| IBIS file stm32f373_378_383_lqfp100.ibs
[IBIS ver] 4.2
[File name] stm32f373_378_383_lqfp100.ibs
[File Rev] 1.0
[Date]  29-09-2025
[Source] Data Created at STMicroelectronics
[Notes]  File originated from ELDO simulations.
[Disclaimer]  This information is for modeling purpose only and is
   not guaranted. The information is subject to change without
   notice.
[Copyright] Copyright 2025 STMicroelectronics Inc.
|   Component stm32f373_378_383_lqfp100
[Component] stm32f373_378_383_lqfp100
[Manufacturer] STMicroelectronics
[Package]
| variable   typ   min   max
R_pkg  0  NA  NA
L_pkg  0  NA  NA
C_pkg  0  NA  NA
[Pin]   signal_name   model_name R_pin  L_pin C_pin
1 PE2 io8p_sudq_ft 0.132430474 7.03397E-09 1.35E-13
2 PE3 io8p_sudq_ft 0.133347678 6.76535E-09 1.95E-14
3 PE4 io8p_sudq_ft 0.12897311 6.4945E-09 1.04E-14
4 PE5 io8p_sudq_ft 0.125344562 6.20552E-09 5.24E-15
5 PE6 io8p_sudq_tc_v33 0.120515446 5.99116E-09 7.82E-15
6 VBAT POWER 0.12047071 5.94998E-09 6.53E-15
7 PC13 io8p_sudq_tc_v33 0.117880646 5.78336E-09 6.23E-15
8 PC14-OSC32_IN io8p_sudq_tc_v33 0.117278614 5.65387E-09 3.11E-15
9 PC15-OSC32_OUT io8p_sudq_tc_v33 0.11554812 5.54782E-09 1.39E-15
10 PF9 io8p_sudq_ft 0.114995632 5.4344E-09 2.92E-15
11 PF10 io8p_sudq_ft 0.112975638 5.2963E-09 3.56E-15
12 PF0-OSC_IN io8p_wsudqh_i2c_ft 0.111323436 5.23061E-09 4.78E-15
13 PF1-OSC_OUT io8p_wsudqh_i2c_ft 0.109216856 5.14191E-09 8.66E-15
14 NRST ioreset_tc_v33 0.11066442 5.17991E-09 9.03E-15
15 PC0 io8p_sudq_ft 0.110607546 5.19248E-09 7.98E-15
16 PC1 io8p_sudq_ft 0.111326184 5.25166E-09 1.03E-14
17 PC2 io8p_sudq_ft 0.11442005 5.34504E-09 7E-15
18 PC3 io8p_sudq_ft 0.114363236 5.45423E-09 8.65E-15
19 PF2 io8p_sudq_ft 0.117563732 5.62144E-09 7.825E-15
20 VSSA/VREF- GND 0.119904688 5.80037E-09 2.29E-16
21 VDDA POWER 0.122311852 5.96269E-09 1.05E-15
22 VREF+ POWER 0.125384354 6.18685E-09 8.12E-16
23 PA0-WKUP1 io8p_sudq_ft 0.129702038 6.48502E-09 3.82E-15
24 PA1 io8p_sudq_ft 0.13229018 6.71495E-09 6.8E-15
25 PA2 io8p_sudq_ft 0.132955142 7.01353E-09 1.67E-14
26 PA3 io8p_sudq_ft 0.13394318 7.04988E-09 1.75E-14
27 PF4 io8p_sudq_ft 0.13495773 6.80443E-09 1.27E-14
28 VDD POWER 0.130511464 6.52834E-09 9.83E-15
29 PA4 io8p_sudq_ft 0.1253867 6.24489E-09 6.07E-15
30 PA5 io8p_sudq_ft 0.124988978 6.10766E-09 5.77E-16
31 PA6 io8p_sudq_ft 0.121784338 5.89035E-09 1.52E-15
32 PA7 io8p_sudq_ft 0.119149388 5.71642E-09 5.44E-15
33 PC4 io8p_sudq_ft 0.116374808 5.55629E-09 4.1E-15
34 PC5 io8p_sudq_ft 0.113278606 5.41493E-09 3.69E-15
35 PB0 io8p_sudq_ft 0.112726654 5.35765E-09 3.895E-15
36 PB1 io8p_sudq_ft 0.112271006 5.27162E-09 1.66E-15
37 PB2 io8p_sudq_ft 0.111816114 5.23836E-09 7.92E-15
38 PE7 io8p_sudq_ft 0.110998514 5.1839E-09 9.9E-15
39 PE8 io8p_sudq_ft 0.114588522 5.29925E-09 7.91E-15
40 PE9 io8p_sudq_ft 0.114461118 5.33298E-09 7.94E-15
41 PE10 io8p_sudq_ft 0.11535023 5.42422E-09 4.18E-15
42 PE11 io8p_sudq_ft 0.116979452 5.53296E-09 6.06E-15
43 PE12 io8p_sudq_ft 0.120184998 5.69823E-09 5.12E-15
44 PE13 io8p_sudq_ft 0.12258702 5.87093E-09 4.74E-15
45 PE14 io8p_sudq_ft 0.126303358 6.06896E-09 1.16E-14
46 PE15 io8p_sudq_ft 0.129714658 6.27741E-09 9.91E-15
47 PB10 io8p_sudq_ft 0.133373154 6.50819E-09 5.08E-15
48 VREFSD- GND 0.137888146 6.85669E-09 5.47E-15
49 VSSSD GND 0.131554082 6.80212E-09 4.18E-15
50 VDDSD12 POWER 0.132347744 7.042E-09 1.19E-14
51 VDDSD3 POWER 0.131767814 7.00793E-09 1.62E-14
52 VREFSD+ POWER 0.131784366 6.75141E-09 2.15E-15
53 PB14 io8p_sudq_ft 0.129150704 6.4828E-09 9.175E-15
54 PB15 io8p_sudq_ft 0.12519135 6.20179E-09 5.6625E-15
55 PD8 io8p_sudq_ft 0.121530258 5.98564E-09 3.69E-15
56 PD9 io8p_sudq_ft 0.11887369 5.8072E-09 7.43E-15
57 PD10 io8p_sudq_ft 0.11586992 5.63548E-09 1.06E-14
58 PD11 io8p_sudq_ft 0.113225758 5.47094E-09 5.76E-15
59 PD12 io8p_sudq_ft 0.111781608 5.35435E-09 6.53E-15
60 PD13 io8p_sudq_ft 0.110712606 5.27649E-09 1.14E-14
61 PD14 io8p_sudq_ft 0.110051596 5.20449E-09 1.32E-14
62 PD15 io8p_sudq_ft 0.10995365 5.1798E-09 1.46E-14
63 PC6 io8p_sudq_ft 0.1097803 5.15375E-09 7.25E-15
64 PC7 io8p_sudq_ft 0.112445854 5.25828E-09 3.59E-16
65 PC8 io8p_sudq_ft 0.113595842 5.33176E-09 6.58E-16
66 PC9 io8p_sudq_ft 0.115707136 5.46645E-09 5.085E-16
67 PA8 io8p_sudq_ft 0.116952062 5.5984E-09 5.8325E-16
68 PA9 io8p_wsudqh_i2c_ft 0.11904328 5.76171E-09 5.45875E-16
69 PA10 io8p_wsudqh_i2c_ft 0.120673854 5.87972E-09 1.39E-14
70 PA11 io8usb_lv_ft 0.124658692 6.10781E-09 2.5E-14
71 PA12 io8usb_lv_ft 0.124406978 6.16144E-09 3.99E-14
72 PA13 io8p_sudq_ft 0.130155984 6.40391E-09 3.02E-13
73 PF6 io8p_wsudqh_i2c_ft 0.135109698 6.82357E-09 1.55E-13
74 VSS GND 0.139401952 7.07731E-09 1.55E-13
75 VDD POWER 0.133554014 7.05568E-09 3.9E-14
76 PA14 io8p_wsudqh_i2c_ft 0.135294596 7.10432E-09 1.63E-14
77 PA15 io8p_wsudqh_i2c_ft 0.132513704 6.8361E-09 9.76E-15
78 PC10 io8p_sudq_ft 0.133481516 6.64112E-09 9.3E-15
79 PC11 io8p_sudq_ft 0.12836612 6.34148E-09 5.42E-15
80 PC12 io8p_sudq_ft 0.124282386 6.09211E-09 1.18E-15
81 PD0 io8p_sudq_ft 0.121841172 5.91673E-09 5.46E-15
82 PD1 io8p_sudq_ft 0.118487054 5.72844E-09 7E-15
83 PD2 io8p_sudq_ft 0.117180194 5.57316E-09 6.06E-15
84 PD3 io8p_sudq_ft 0.11350052 5.42154E-09 5.45E-15
85 PD4 io8p_sudq_ft 0.113789098 5.34394E-09 5.29E-16
86 PD5 io8p_sudq_ft 0.110805858 5.25639E-09 2.9895E-15
87 PD6 io8p_sudq_ft 0.110442376 5.2462E-09 2.06E-15
88 PD7 io8p_sudq_ft 0.111525472 5.17788E-09 5.68E-15
89 PB3 io8p_sudq_ft 0.11114441 5.22307E-09 9.91E-15
90 PB4 io8p_sudq_ft 0.113222316 5.31007E-09 9.05E-15
91 PB5 io8p_sudq_ft 0.113322882 5.40053E-09 1.29E-14
92 PB6 io8p_wsudqh_i2c_ft 0.1158486 5.51866E-09 1.26E-14
93 PB7 io8p_wsudqh_i2c_ft 0.117577758 5.67321E-09 6.14E-15
94 BOOT0 vpp_test_hv 0.1189821 5.80207E-09 9.37E-15
95 PB8 io8p_wsudqh_i2c_ft 0.121885942 5.96185E-09 7.755E-15
96 PB9 io8p_wsudqh_i2c_ft 0.126275558 6.15795E-09 8.5625E-15
97 PE0 io8p_sudq_ft 0.128749356 6.36737E-09 8.15875E-15
98 PE1 io8p_sudq_ft 0.13328845 6.70016E-09 1.03E-15
99 VSS GND 0.13223018 6.84396E-09 4.41E-15
100 VDD POWER 0.132277204 7.05248E-09 1.71E-14
[Model Selector] io8p_sudq_ft
io8p01_sudq_ft_pd_lv  "SPEED01 2P0V, PD=40kOhm"
io8p01_sudq_ft_pu_lv  "SPEED01 2P0V, PU=40kOhm"
io8p01_sudq_ft_lv  "SPEED01 2P0V"
io8p10_sudq_ft_pd_lv  "SPEED10 2P0V, PD=40kOhm"
io8p10_sudq_ft_pu_lv  "SPEED10 2P0V, PU=40kOhm"
io8p10_sudq_ft_lv  "SPEED10 2P0V"
io8p11_sudq_ft_pd_lv  "SPEED11 2P0V, PD=40kOhm"
io8p11_sudq_ft_pu_lv  "SPEED11 2P0V, PU=40kOhm"
io8p11_sudq_ft_lv  "SPEED11 2P0V"
io8p01_sudq_ft_pd  "SPEED01, PD=40kOhm"
io8p01_sudq_ft_pu  "SPEED01, PU=40kOhm"
io8p01_sudq_ft  "SPEED01"
io8p10_sudq_ft_pd  "SPEED10, PD=40kOhm"
io8p10_sudq_ft_pu  "SPEED10, PU=40kOhm"
io8p10_sudq_ft  "SPEED10"
io8p11_sudq_ft_pd  "SPEED11, PD=40kOhm"
io8p11_sudq_ft_pu  "SPEED11, PU=40kOhm"
io8p11_sudq_ft  "SPEED11"
[Model Selector] io8p_sudq_tc_v33
io8p01_sudq_tc_v33_pd_lv  "SPEED01 2P0V, PD=40kOhm"
io8p01_sudq_tc_v33_pu_lv  "SPEED01 2P0V, PU=40kOhm"
io8p01_sudq_tc_v33_lv  "SPEED01 2P0V"
io8p10_sudq_tc_v33_pd_lv  "SPEED10 2P0V, PD=40kOhm"
io8p10_sudq_tc_v33_pu_lv  "SPEED10 2P0V, PU=40kOhm"
io8p10_sudq_tc_v33_lv  "SPEED10 2P0V"
io8p11_sudq_tc_v33_pd_lv  "SPEED11 2P0V, PD=40kOhm"
io8p11_sudq_tc_v33_pu_lv  "SPEED11 2P0V, PU=40kOhm"
io8p11_sudq_tc_v33_lv  "SPEED11 2P0V"
io8p01_sudq_tc_v33_pd  "SPEED01, PD=40kOhm"
io8p01_sudq_tc_v33_pu  "SPEED01, PU=40kOhm"
io8p01_sudq_tc_v33  "SPEED01"
io8p10_sudq_tc_v33_pd  "SPEED10, PD=40kOhm"
io8p10_sudq_tc_v33_pu  "SPEED10, PU=40kOhm"
io8p10_sudq_tc_v33  "SPEED10"
io8p11_sudq_tc_v33_pd  "SPEED11, PD=40kOhm"
io8p11_sudq_tc_v33_pu  "SPEED11, PU=40kOhm"
io8p11_sudq_tc_v33  "SPEED11"
[Model Selector] io8p_wsudqh_i2c_ft
io8p_wsudqh_i2c_ft_lv_pd  "General purpose IO with I2C capability on. 5V tolerant. 1.8V range with pull down"
io8p_wsudqh_i2c_ft_lv_pu  "General purpose IO with I2C capability on. 5V tolerant. 1.8V range with pull up"
io8p_wsudqh_i2c_ft_lv  "General purpose IO with I2C capability on. 5V tolerant. 1.8V range"
io8p_wsudqh_i2c_ft_pd  "General purpose IO with I2C capability on. 5V tolerant. 3.3V range with pull down"
io8p_wsudqh_i2c_ft_pu  "General purpose IO with I2C capability on. 5V tolerant. 3.3V range with pull up"
io8p_wsudqh_i2c_ft_i2c  "General purpose IO with I2C capability on. 5V tolerant. 3.3V range"
[Model Selector] io8usb_lv_ft
io8usb_dpdn_lv_ft_pd  "FS USB DP/DN IO + PD=40kOhm"
io8usb_dpdn_lv_ft_pu  "FS USB DP/DN IO + PU=40kOhm"
io8usb_dpdn_lv_ft  "FS USB DP/DN IO"
io8p01_lv_ft_pd_lv  "SPEED01 2P0V, PD=40kOhm"
io8p01_lv_ft_pu_lv  "SPEED01 2P0V, PU=40kOhm"
io8p01_lv_ft_lv  "SPEED01 2P0V"
io8p10_lv_ft_pd_lv  "SPEED10 2P0V, PD=40kOhm"
io8p10_lv_ft_pu_lv  "SPEED10 2P0V, PU=40kOhm"
io8p10_lv_ft_lv  "SPEED10 2P0V"
io8p11_lv_ft_pd_lv  "SPEED11 2P0V, PD=40kOhm"
io8p11_lv_ft_pu_lv  "SPEED11 2P0V, PU=40kOhm"
io8p11_lv_ft_lv  "SPEED11 2P0V"
io8p01_lv_ft_pd  "SPEED01, PD=40kOhm"
io8p01_lv_ft_pu  "SPEED01, PU=40kOhm"
io8p01_lv_ft  "SPEED01"
io8p10_lv_ft_pd  "SPEED10, PD=40kOhm"
io8p10_lv_ft_pu  "SPEED10, PU=40kOhm"
io8p10_lv_ft  "SPEED10"
io8p11_lv_ft_pd  "SPEED11, PD=40kOhm"
io8p11_lv_ft_pu  "SPEED11, PU=40kOhm"
io8p11_lv_ft  "SPEED11"
[Model Selector] ioreset_tc_v33
ioreset_tc_v33_pu_lv  "IORESET 2V + PU=40kOhm"
ioreset_tc_v33_nopu_lv  "IORESET 2V"
ioreset_tc_v33_pu  "IORESET + PU=40kOhm"
ioreset_tc_v33_nopu  "IORESET"
[Model Selector] vpp_test_hv
vpp_test_hv_3p3  "Input Buffer"
vpp_test_hv_2p4  "Input Buffer 2P0V"
| Models and submodels in the file (69): io8p01_sudq_ft_pd_lv (I/O), io8p01_sudq_ft_pu_lv (I/O), io8p01_sudq_ft_lv (I/O), io8p10_sudq_ft_pd_lv (I/O), io8p10_sudq_ft_pu_lv (I/O), io8p10_sudq_ft_lv (I/O), io8p11_sudq_ft_pd_lv (I/O), io8p11_sudq_ft_pu_lv (I/O), io8p11_sudq_ft_lv (I/O), io8p01_sudq_ft_pd (I/O), io8p01_sudq_ft_pu (I/O), io8p01_sudq_ft (I/O), io8p10_sudq_ft_pd (I/O), io8p10_sudq_ft_pu (I/O), io8p10_sudq_ft (I/O), io8p11_sudq_ft_pd (I/O), io8p11_sudq_ft_pu (I/O), io8p11_sudq_ft (I/O), io8p01_sudq_tc_v33_pd_lv (I/O), io8p01_sudq_tc_v33_pu_lv (I/O), io8p01_sudq_tc_v33_lv (I/O), io8p10_sudq_tc_v33_pd_lv (I/O), io8p10_sudq_tc_v33_pu_lv (I/O), io8p10_sudq_tc_v33_lv (I/O), io8p11_sudq_tc_v33_pd_lv (I/O), io8p11_sudq_tc_v33_pu_lv (I/O), io8p11_sudq_tc_v33_lv (I/O), io8p01_sudq_tc_v33_pd (I/O), io8p01_sudq_tc_v33_pu (I/O), io8p01_sudq_tc_v33 (I/O), io8p10_sudq_tc_v33_pd (I/O), io8p10_sudq_tc_v33_pu (I/O), io8p10_sudq_tc_v33 (I/O), io8p11_sudq_tc_v33_pd (I/O), io8p11_sudq_tc_v33_pu (I/O), io8p11_sudq_tc_v33 (I/O), io8p_wsudqh_i2c_ft_lv_pd (I/O), io8p_wsudqh_i2c_ft_lv_pu (I/O), io8p_wsudqh_i2c_ft_lv (I/O), io8p_wsudqh_i2c_ft_pd (I/O), io8p_wsudqh_i2c_ft_pu (I/O), io8p_wsudqh_i2c_ft_i2c (I/O), io8usb_dpdn_lv_ft_pd (I/O), io8usb_dpdn_lv_ft_pu (I/O), io8usb_dpdn_lv_ft (I/O), io8p01_lv_ft_pd_lv (I/O), io8p01_lv_ft_pu_lv (I/O), io8p01_lv_ft_lv (I/O), io8p10_lv_ft_pd_lv (I/O), io8p10_lv_ft_pu_lv (I/O), io8p10_lv_ft_lv (I/O), io8p11_lv_ft_pd_lv (I/O), io8p11_lv_ft_pu_lv (I/O), io8p11_lv_ft_lv (I/O), io8p01_lv_ft_pd (I/O), io8p01_lv_ft_pu (I/O), io8p01_lv_ft (I/O), io8p10_lv_ft_pd (I/O), io8p10_lv_ft_pu (I/O), io8p10_lv_ft (I/O), io8p11_lv_ft_pd (I/O), io8p11_lv_ft_pu (I/O), io8p11_lv_ft (I/O), ioreset_tc_v33_pu_lv (I/O_open_drain), ioreset_tc_v33_nopu_lv (I/O_open_drain), ioreset_tc_v33_pu (I/O_open_drain), ioreset_tc_v33_nopu (I/O_open_drain), vpp_test_hv_2p4 (Input), vpp_test_hv_3p3 (Input)
